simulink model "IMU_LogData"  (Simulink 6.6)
settings: Solver=FixedStepDiscrete  StartTime=0.0  StopTime=10.0  FixedStep=0.001  RelTol=1e-3
undefined symbols (not defined in the file or in its folder): bits, hex2dec
libraries: dsPICdrivers x31, simulink x13

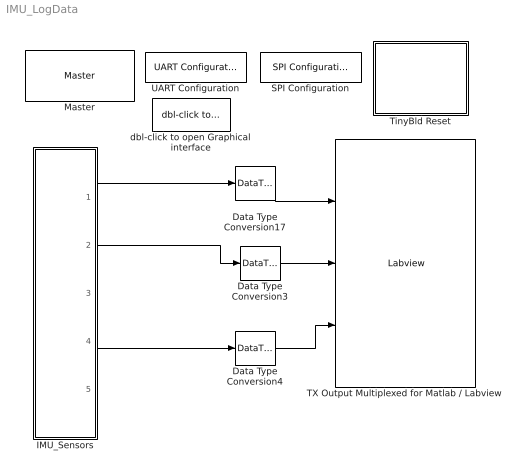
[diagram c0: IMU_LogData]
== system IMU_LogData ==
  Data Type Conversion17 : DataTypeConversion  OutDataTypeMode=int16  OutScaling="[ (80/(2048*2^4))  0]"  ConvertRealWorld=Stored Integer (SI)
  Data Type Conversion3 : DataTypeConversion  OutDataTypeMode=int16  OutScaling="[ (80/(2048*2^4))  0]"  ConvertRealWorld=Stored Integer (SI)
  Data Type Conversion4 : DataTypeConversion  OutDataTypeMode=int16  OutScaling="[ (80/(2048*2^4))  0]"  ConvertRealWorld=Stored Integer (SI)
  IMU_Sensors : Subsystem
  Master : dsPICdrivers/Master  Tag=dsPIC_MASTER  Priority=1  TimeStepType=Timer1  picType=30f4012  fcy=20e6  Quartz_33f=5e6  PLLActive_33f=off  fcyDesired_33f=0  tmr1="[1  20000  0]"  tmr1Info="Time Step : 0.001  ;   Error : 0%  PR1=20000"  tmr2345="[0  0  0  0]"  tmr2345cfg=[-1 -1 -1 -1]  IOautoConf=on  typePort="[ 0   0   0   0   0   0   0   0   0   0   0   0   0   0   0   0   0   0   0   0   0   0   0   0   0   0   0   0   0   0   0   0   0   0   0   0   0   0   0   0   0   0   0   0   0   5   4   0   0   0   0   0   0   0   0   0   0   0   0   0   0   0   0   0   0   0   0  10   0  10   0   0  17   0   0   0   0   0   0   0   0   0  14  15   0   0   0   0   0   0   0   0   0   0   0   0   0   0   0   0 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"  TRIS="[ 65535  65535  65535  65535  65495  65535  65535 ]"  ADPCFG=0  MasterBusyPort=None  MasterOverloadPort=None  FOSC=XT_PLL8  TempProtection_33f=TEMP_ON  FPBOR=PBOR_OFF  PWRT=PWRT_4  MCLR=MCLR_DIS  PowerSave=off
  SPI Configuration : dsPICdrivers/SPI PORT/SPI Configuration  Tag=dsPIC_config_SPI  Priority=2  Frame_Enable=0  Frame_Sync=0  SPI=1  MODE=MASTER  USER_SCALER=12  StartEnable=Enable  SDO_EN=on  DATA_LENGTH=16 bits  SS_EN=off  SMP=Middle of bit  CKP=high  CKE=Idle to Active  Status=Fsck= Not Available
  TX Output Multiplexed for Matlab / Labview : dsPICdrivers/Serial PORT/TX Output Multiplexed for Matlab // Labview  Tag=dsPIC_TX_Multiplexed  Priority=5  UART=1  CleverSpreadingChk=on  CleverSpreading=1  CHANNEL=[0 1 2 ]  BUFFERSIZE=16  CHANNELBLOCKED=[]  CHANNELBLOCKED_BITEWISE=0  Status=OK
  TinyBld Reset : Subsystem  AncestorBlock=dsPICdrivers/OTHERS/TinyBld Reset
  UART Configuration : dsPICdrivers/Serial PORT/UART Configuration  Tag=dsPIC_config_UART  Priority=2  UART=1  proposed_BAUD=115200  ALT_TX_RX=on  TXInterruptPri=1  InterruptTxWhen=on TxBUF becoming empty  TXEN=on  RXInterruptPri=1  BAUD=115200  UxBRG=10  Info="UxBRG = 10   ||  Real Baud : 113636   ||  % error : -1.3573  ||  max 11.3636 Bytes / Step"  RealBaud=0
  dbl-click to open Graphical interface : dsPICdrivers/Serial PORT/dbl-click to open Graphical interface  SystemSampleTime=-1
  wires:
  IMU_Sensors/1(AccelX) -> Data Type Conversion17/1
  IMU_Sensors/4(AccelZ) -> Data Type Conversion4/1
  IMU_Sensors/2(GyroY) -> Data Type Conversion3/1
  Data Type Conversion17/1 -> TX Output Multiplexed for Matlab / Labview/1
  Data Type Conversion3/1 -> TX Output Multiplexed for Matlab / Labview/2
  Data Type Conversion4/1 -> TX Output Multiplexed for Matlab / Labview/3

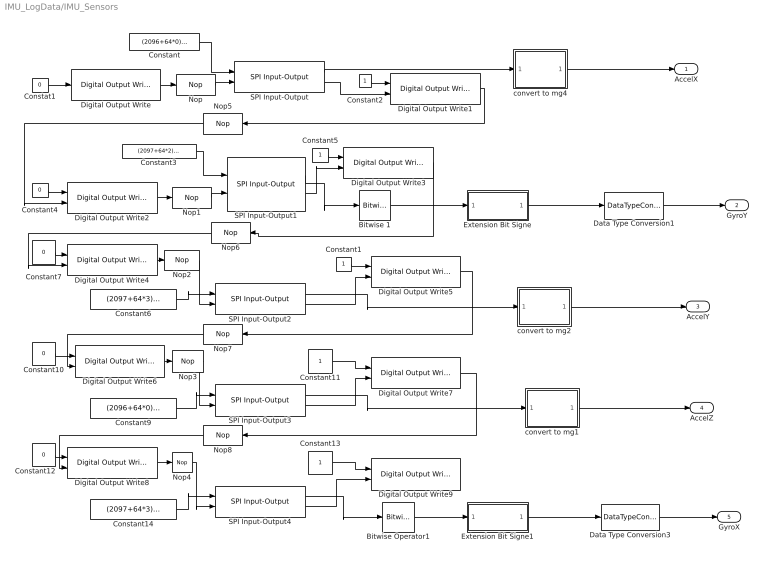
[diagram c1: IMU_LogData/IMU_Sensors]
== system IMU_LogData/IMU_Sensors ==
  Bitwise Operator1 : simulink/Logic and Bit Operations/Bitwise Operator  logicop=AND  UseBitMask=on  BitMask=hex2dec('0FFF')  BitMaskRealWorld=Stored Integer
  Bitwise 1 : simulink/Logic and Bit Operations/Bitwise Operator  logicop=AND  UseBitMask=on  BitMask=hex2dec('0FFF')  BitMaskRealWorld=Stored Integer
  Constant : Constant  Value=(2096+64*0)*16  OutDataTypeMode=uint16  SampleTime=-1
  Constant{1..2,5,11,13} (5 alike) : Constant  OutDataTypeMode=boolean  SampleTime=-1
  Constant{4,7,10,12} (4 alike) : Constant  Value=0  OutDataTypeMode=boolean  SampleTime=-1
  Constant14 : Constant  Value=(2097+64*3)*16  OutDataTypeMode=uint16  SampleTime=-1
  Constant3 : Constant  Value=(2097+64*2)*16  VectorParams1D=off  OutDataTypeMode=uint16  SampleTime=-1
  Constant6 : Constant  Value=(2097+64*3)*16  OutDataTypeMode=uint16  SampleTime=-1
  Constant9 : Constant  Value=(2096+64*0)*16  OutDataTypeMode=uint16  SampleTime=-1
  Constat1 : Constant  Value=0  OutDataTypeMode=boolean  SampleTime=-1
  Data Type Conversion1 : DataTypeConversion  OutDataTypeMode=Specify via dialog  OutDataType=sfix(12)  OutScaling="[ (160/4096)  0]"  ConvertRealWorld=Stored Integer (SI)
  Data Type Conversion3 : DataTypeConversion  OutDataTypeMode=Specify via dialog  OutDataType=sfix(12)  OutScaling="[ (160/4096)  0]"  ConvertRealWorld=Stored Integer (SI)
  Digital Output Write : dsPICdrivers/Digital I//O/Digital Output Write  Tag=dsPIC_Digital_Output  Priority=5  PORT=E  Pin=5  OrderingInOutPopup=Output
  Digital Output Write{1..5} (5 alike) : dsPICdrivers/Digital I//O/Digital Output Write  Tag=dsPIC_Digital_Output  Priority=5  PORT=E  Pin=5  OrderingInOutPopup=Input & Output
  Digital Output Write6 : dsPICdrivers/Digital I//O/Digital Output Write  Tag=dsPIC_Digital_Output  Priority=5  PORT=E  Pin=3  OrderingInOutPopup=Input & Output
  Digital Output Write7 : dsPICdrivers/Digital I//O/Digital Output Write  Tag=dsPIC_Digital_Output  Priority=5  PORT=E  Pin=3  OrderingInOutPopup=Input & Output
  Digital Output Write8 : dsPICdrivers/Digital I//O/Digital Output Write  Tag=dsPIC_Digital_Output  Priority=5  PORT=E  Pin=3  OrderingInOutPopup=Input & Output
  Digital Output Write9 : dsPICdrivers/Digital I//O/Digital Output Write  Tag=dsPIC_Digital_Output  Priority=5  PORT=E  Pin=3  OrderingInOutPopup=Input
  Extension Bit Signe : Subsystem  TreatAsAtomicUnit=on
  Extension Bit Signe1 : Subsystem  TreatAsAtomicUnit=on
  Nop{,1..4} (5 alike) : dsPICdrivers/OTHERS/Nop  Tag=dsPIC_Reset  NbrNop=5
  Nop{5..8} (4 alike) : dsPICdrivers/OTHERS/Nop  Tag=dsPIC_Reset  Orientation=left  NbrNop=5
  SPI Input-Output{,1..4} (5 alike) : dsPICdrivers/SPI PORT/SPI Input-Output  Tag=dsPIC_SPI  SPI=1  INPUT=on  RESET_INPUT=off  OUTPUT=on  SPECIAL_SPI=Always Enable  DATA_LENGTH=16 bits  WAIT_INPUTDATA=on  OrderingInOutPopup=Input & Output
  convert to mg1 : Subsystem  TreatAsAtomicUnit=on
  convert to mg2 : Subsystem  TreatAsAtomicUnit=on
  convert to mg4 : Subsystem  TreatAsAtomicUnit=on
  AccelX : Outport
  GyroY : Outport  Port=2
  AccelY : Outport  Port=3
  AccelZ : Outport  Port=4
  GyroX : Outport  Port=5
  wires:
  Constant2/1 -> Digital Output Write1/1
  Constat1/1 -> Digital Output Write/1
  Constant5/1 -> Digital Output Write3/1
  Constant4/1 -> Digital Output Write2/1
  Digital Output Write1/1 -> Nop5/1
  Constant1/1 -> Digital Output Write5/1
  Constant11/1 -> Digital Output Write7/1
  Constant10/1 -> Digital Output Write6/1
  Digital Output Write5/1 -> Nop7/1
  Constant13/1 -> Digital Output Write9/1
  Constant12/1 -> Digital Output Write8/1
  Digital Output Write7/1 -> Nop8/1
  Digital Output Write/1 -> Nop/1
  Constant/1 -> SPI Input-Output/1
  SPI Input-Output/2 -> Digital Output Write1/2
  SPI Input-Output/1 -> convert to mg4/1(In1)
  Constant3/1 -> SPI Input-Output1/1
  Digital Output Write2/1 -> Nop1/1
  SPI Input-Output1/2 -> Digital Output Write3/2
  SPI Input-Output1/1 -> Bitwise 1/1
  Constant7/1 -> Digital Output Write4/1
  Digital Output Write4/1 -> Nop2/1
  Constant6/1 -> SPI Input-Output2/1
  SPI Input-Output2/1 -> convert to mg2/1(In1)
  SPI Input-Output2/2 -> Digital Output Write5/2
  Digital Output Write6/1 -> Nop3/1
  Constant9/1 -> SPI Input-Output3/1
  SPI Input-Output3/1 -> convert to mg1/1(In1)
  SPI Input-Output3/2 -> Digital Output Write7/2
  Constant14/1 -> SPI Input-Output4/1
  Digital Output Write8/1 -> Nop4/1
  SPI Input-Output4/1 -> Bitwise Operator1/1
  SPI Input-Output4/2 -> Digital Output Write9/2
  convert to mg4/1(Out1) -> AccelX/1
  Data Type Conversion1/1 -> GyroY/1
  Nop/1 -> SPI Input-Output/2
  Nop1/1 -> SPI Input-Output1/2
  Nop2/1 -> SPI Input-Output2/2
  Nop3/1 -> SPI Input-Output3/2
  Nop4/1 -> SPI Input-Output4/2
  Nop5/1 -> Digital Output Write2/2
  Nop6/1 -> Digital Output Write4/2
  Nop7/1 -> Digital Output Write6/2
  Nop8/1 -> Digital Output Write8/2
  Bitwise Operator1/1 -> Extension Bit Signe1/1(In1)
  Data Type Conversion3/1 -> GyroX/1
  convert to mg1/1(Out1) -> AccelZ/1
  convert to mg2/1(Out1) -> AccelY/1
  Digital Output Write3/1 -> Nop6/1
  Bitwise 1/1 -> Extension Bit Signe/1(In1)
  Extension Bit Signe/1(Out1) -> Data Type Conversion1/1
  Extension Bit Signe1/1(Out1) -> Data Type Conversion3/1

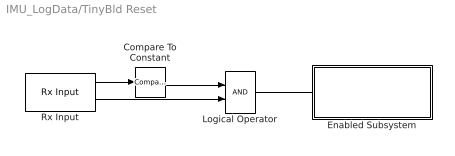
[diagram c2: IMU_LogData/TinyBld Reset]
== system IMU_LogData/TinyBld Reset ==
  Compare To Constant : simulink/Logic and Bit Operations/Compare To Constant  SystemSampleTime=-1  relop===  const=55  LogicOutDataTypeMode=boolean  ZeroCross=off
  Enabled Subsystem : Subsystem  Orientation=up  TreatAsAtomicUnit=on
  Logical Operator : Logic  AllPortsSameDT=off  OutDataTypeMode=Boolean
  Rx Input : dsPICdrivers/Serial PORT/Rx Input  Tag=dsPIC_RX  Priority=5  UART=1  SampleTime=.01  BlockingFctChk=off  OutputDefault=0  IsPresentFlagChk=on
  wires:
  Rx Input/1 -> Compare To Constant/1
  Compare To Constant/1 -> Logical Operator/1
  Rx Input/2 -> Logical Operator/2
  Logical Operator/1 -> Enabled Subsystem/Enable

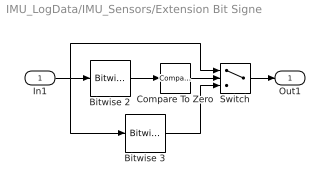
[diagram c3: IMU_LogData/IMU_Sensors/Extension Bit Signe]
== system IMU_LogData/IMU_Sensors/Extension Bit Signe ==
  In1 : Inport
  Bitwise 2 : simulink/Logic and Bit Operations/Bitwise Operator  logicop=AND  UseBitMask=on  BitMask=2^11  BitMaskRealWorld=Stored Integer
  Bitwise 3 : simulink/Logic and Bit Operations/Bitwise Operator  logicop=OR  UseBitMask=on  BitMask=hex2dec('F000')  BitMaskRealWorld=Stored Integer
  Compare To Zero : simulink/Logic and Bit Operations/Compare To Zero  SystemSampleTime=-1  relop===  LogicOutDataTypeMode=boolean  ZeroCross=off
  Switch : Switch  Criteria=u2 ~= 0
  Out1 : Outport
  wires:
  In1/1 -> Bitwise 3/1, Switch/1, Bitwise 2/1
  Bitwise 2/1 -> Compare To Zero/1
  Compare To Zero/1 -> Switch/2
  Bitwise 3/1 -> Switch/3
  Switch/1 -> Out1/1

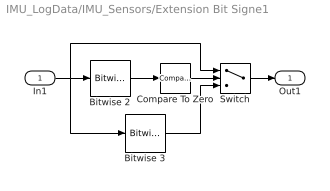
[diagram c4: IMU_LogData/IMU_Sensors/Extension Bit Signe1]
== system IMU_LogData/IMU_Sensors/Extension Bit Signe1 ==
  In1 : Inport
  Bitwise 2 : simulink/Logic and Bit Operations/Bitwise Operator  logicop=AND  UseBitMask=on  BitMask=2^11  BitMaskRealWorld=Stored Integer
  Bitwise 3 : simulink/Logic and Bit Operations/Bitwise Operator  logicop=OR  UseBitMask=on  BitMask=hex2dec('F000')  BitMaskRealWorld=Stored Integer
  Compare To Zero : simulink/Logic and Bit Operations/Compare To Zero  SystemSampleTime=-1  relop===  LogicOutDataTypeMode=boolean  ZeroCross=off
  Switch : Switch  Criteria=u2 ~= 0
  Out1 : Outport
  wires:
  Switch/1 -> Out1/1
  Bitwise 3/1 -> Switch/3
  Compare To Zero/1 -> Switch/2
  Bitwise 2/1 -> Compare To Zero/1
  In1/1 -> Bitwise 2/1, Switch/1, Bitwise 3/1

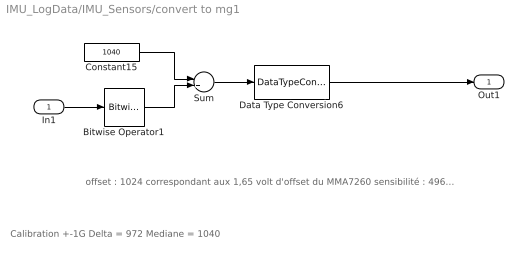
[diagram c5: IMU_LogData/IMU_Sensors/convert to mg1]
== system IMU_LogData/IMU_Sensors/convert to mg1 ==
  note: offset : 1024 correspondant aux 1,65 volt d'offset du MMA7260 sensibilité : 496.484848 / g ==> (2mg) Le composant est alimenté en 2.5V au lieu de 3.3V
  note: Calibration +-1G Delta = 972 Mediane = 1040
  In1 : Inport
  Bitwise Operator1 : simulink/Logic and Bit Operations/Bitwise Operator  logicop=AND  UseBitMask=on  BitMask=4095  BitMaskRealWorld=Stored Integer
  Constant15 : Constant  Value=1040  OutDataTypeMode=int16  SampleTime=-1
  Data Type Conversion6 : DataTypeConversion  OutDataTypeMode=Specify via dialog  OutDataType=sfix(12)  OutScaling=[1/486*1000 0]  ConvertRealWorld=Stored Integer (SI)
  Sum : Sum  Inputs=-+  OutDataTypeMode=int16
  Out1 : Outport
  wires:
  In1/1 -> Bitwise Operator1/1
  Data Type Conversion6/1 -> Out1/1
  Constant15/1 -> Sum/1
  Sum/1 -> Data Type Conversion6/1
  Bitwise Operator1/1 -> Sum/2

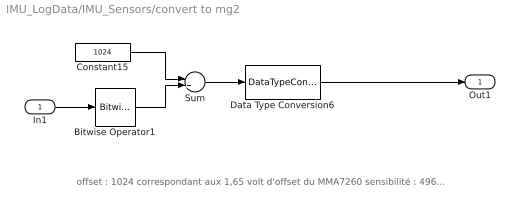
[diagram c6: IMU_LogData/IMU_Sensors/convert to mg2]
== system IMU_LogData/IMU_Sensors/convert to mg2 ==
  note: offset : 1024 correspondant aux 1,65 volt d'offset du MMA7260 sensibilité : 496.484848 / g ==> (2mg) Le composant est alimenté en 2.5V au lieu de 3.3V
  In1 : Inport
  Bitwise Operator1 : simulink/Logic and Bit Operations/Bitwise Operator  logicop=AND  UseBitMask=on  BitMask=4095  BitMaskRealWorld=Stored Integer
  Constant15 : Constant  Value=1024  OutDataTypeMode=int16  SampleTime=-1
  Data Type Conversion6 : DataTypeConversion  OutDataTypeMode=Specify via dialog  OutDataType=sfix(12)  OutScaling=[1/496.484848*1000 0]  ConvertRealWorld=Stored Integer (SI)
  Sum : Sum  Inputs=-+  OutDataTypeMode=int16
  Out1 : Outport
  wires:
  Bitwise Operator1/1 -> Sum/2
  Sum/1 -> Data Type Conversion6/1
  Constant15/1 -> Sum/1
  Data Type Conversion6/1 -> Out1/1
  In1/1 -> Bitwise Operator1/1

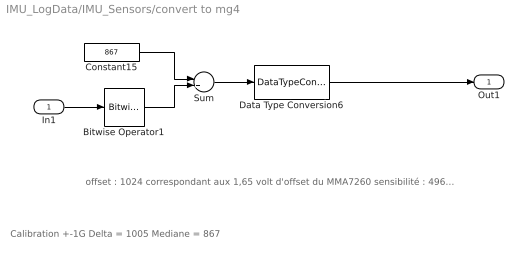
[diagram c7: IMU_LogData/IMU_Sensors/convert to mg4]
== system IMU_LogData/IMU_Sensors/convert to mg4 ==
  note: Calibration +-1G Delta = 1005 Mediane = 867
  note: offset : 1024 correspondant aux 1,65 volt d'offset du MMA7260 sensibilité : 496.484848 / g ==> (2mg) Le composant est alimenté en 2.5V au lieu de 3.3V
  In1 : Inport
  Bitwise Operator1 : simulink/Logic and Bit Operations/Bitwise Operator  logicop=AND  UseBitMask=on  BitMask=4095  BitMaskRealWorld=Stored Integer
  Constant15 : Constant  Value=867  OutDataTypeMode=int16  SampleTime=-1
  Data Type Conversion6 : DataTypeConversion  OutDataTypeMode=Specify via dialog  OutDataType=sfix(12)  OutScaling=[1/502.5*1000 0]  ConvertRealWorld=Stored Integer (SI)
  Sum : Sum  Inputs=-+  OutDataTypeMode=int16
  Out1 : Outport
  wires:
  Bitwise Operator1/1 -> Sum/2
  Sum/1 -> Data Type Conversion6/1
  Constant15/1 -> Sum/1
  Data Type Conversion6/1 -> Out1/1
  In1/1 -> Bitwise Operator1/1

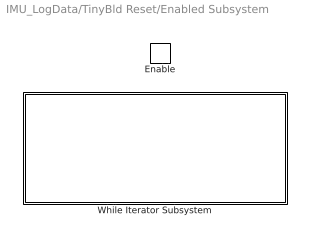
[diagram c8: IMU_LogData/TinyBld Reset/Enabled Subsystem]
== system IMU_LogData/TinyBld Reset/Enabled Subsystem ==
  Enable : EnablePort
  While Iterator Subsystem : Subsystem  TreatAsAtomicUnit=on

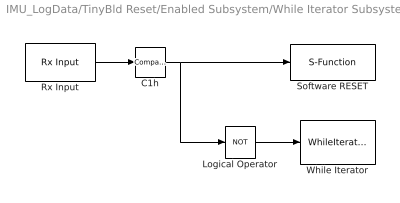
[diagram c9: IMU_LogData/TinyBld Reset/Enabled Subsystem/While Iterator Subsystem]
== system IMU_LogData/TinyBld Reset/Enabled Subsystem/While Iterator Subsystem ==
  C1h : simulink/Logic and Bit Operations/Compare To Constant  SystemSampleTime=-1  relop===  const=66  LogicOutDataTypeMode=boolean  ZeroCross=off
  Logical Operator : Logic  Operator=NOT  AllPortsSameDT=off  OutDataTypeMode=Boolean
  Rx Input : dsPICdrivers/Serial PORT/Rx Input  Tag=dsPIC_RX  Priority=5  UART=1  SampleTime=-1  BlockingFctChk=on  OutputDefault=0  IsPresentFlagChk=off
  Software RESET : S-Function  Tag=dsPIC_Reset  FunctionName=dsPIC_Reset
  While Iterator : WhileIterator  MaxIters=-1  WhileBlockType=do-while  ResetStates=reset
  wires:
  Logical Operator/1 -> While Iterator/1
  Rx Input/1 -> C1h/1
  C1h/1 -> Software RESET/1, Logical Operator/1
